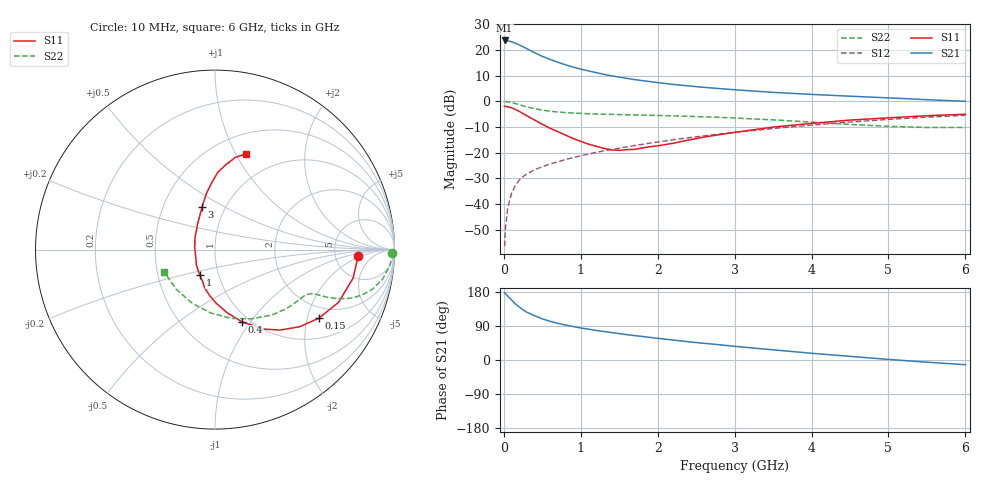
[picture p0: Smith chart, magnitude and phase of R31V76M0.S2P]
! SIEMENS Small Signal Semiconductors
! BFR181
! Si NPN RF Bipolar Junction Transistor in SOT23
! VCE = 1.75 V  IC = 6 mA
! Common Emitter S-Parameters:  May  1996
# GHz  S  MA  R  50
!  f  S11  S21  S12  S22
! GHz  MAG  ANG  MAG  ANG  MAG  ANG  MAG  ANG
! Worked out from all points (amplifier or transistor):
!   36 points, 10 MHz to 6 GHz, reference 50 ohm
!   highest |S21| = 23.7 dB at 10 MHz (marker M1)
!   |S21| within 3 dB of that: start of sweep to 284.3 MHz
!   unconditionally stable (mu >= 1): 930.8 MHz to 2.864 GHz
!   at 250 MHz: K = 0.48, MSG = 25.3 dB, |S12| = -29.3 dB
!   at 1.4 GHz: K = 1.07, MAG = 12.7 dB, |S12| = -18.8 dB
!   at 6 GHz: K = 0.86, MSG = 2.7 dB, |S12| = -5.5 dB
!   S11 on the Smith chart (normalised r, x): 10 MHz: 8.63, -1.66; 150 MHz: 1.61, -2.36; 400 MHz: 0.92, -0.91; 1 GHz: 0.81, -0.24; 3 GHz: 0.78, +0.39; 6 GHz: 0.71, +1.10
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0.01  0.7991 -2.5  15.38 177.7  0.0015 92.9  0.9888 -1.0
0.02  0.7933 -4.9  15.3 175.3  0.0032 77.1  0.9871 -2.2
0.05  0.7854 -11.7  15.13 168.8  0.0084 84.1  0.9771 -5.3
0.1  0.7484 -23.1  14.53 158.4  0.016 78.7  0.9485 -10.0
0.15  0.6937 -33.4  13.61 147.9  0.023 72.8  0.9045 -14.1
0.2  0.6385 -42.3  12.59 140.0  0.029 70.5  0.8609 -16.9
0.25  0.5769 -51.0  11.59 132.2  0.0341 67.4  0.8182 -19.1
0.3  0.5225 -58.0  10.58 126.0  0.0384 66.5  0.7776 -20.6
0.4  0.4309 -69.4  8.888 116.7  0.0466 64.3  0.7178 -22.2
0.5  0.3577 -79.2  7.537 108.5  0.053 63.6  0.6743 -23.1
0.6  0.2989 -88.7  6.578 102.2  0.06 63.9  0.6419 -23.5
0.8  0.2201 -105.2  5.16 92.3  0.0733 64.2  0.6032 -24.0
1  0.1658 -120.6  4.252 84.6  0.0866 65.2  0.5816 -25.1
1.1  0.1464 -131.0  3.923 81.4  0.0938 65.4  0.5734 -25.8
1.3  0.121 -150.3  3.363 75.2  0.1081 65.6  0.5608 -27.3
1.6  0.1146 174.5  2.799 66.9  0.13 65.5  0.5476 -30.2
2.2  0.152 132.5  2.136 52.7  0.1779 63.4  0.5211 -37.9
3  0.2477 107.0  1.682 36.1  0.2476 58.2  0.4729 -51.2
3.5  0.3147 98.9  1.494 26.8  0.2949 53.9  0.4351 -62.4
4.5  0.431 87.9  1.259 9.6  0.3946 43.1  0.3544 -93.5
5.5  0.5249 77.7  1.076 -5.8  0.4913 30.1  0.309 -134.5
6  0.5593 72.3  1.002 -12.4  0.5339 22.9  0.3092 -156.4
